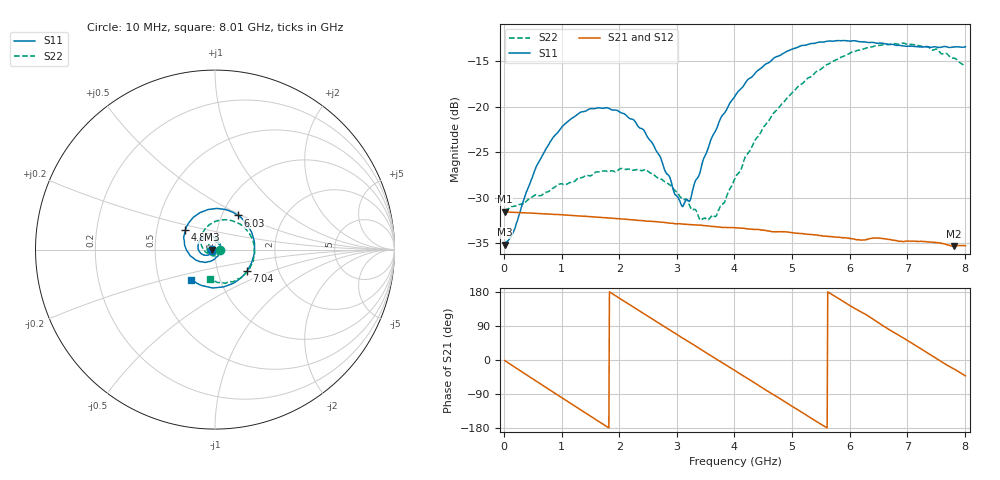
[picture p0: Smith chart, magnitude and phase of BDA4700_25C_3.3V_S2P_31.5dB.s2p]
!Agilent Technologies,E5071B,MY42404982,A.09.10
!Date: Mon Oct 20 18:16:19 2025
!Data & Calibration Information:
!Freq	S11:SOLT2(ON)	S21:SOLT2(ON)	S12:SOLT2(ON)	S22:SOLT2(ON)
# Hz S RI R 50
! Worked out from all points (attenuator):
!   801 points, 10 MHz to 8.01 GHz, reference 50 ohm
!   highest |S21| = -31.55 dB at 10 MHz (marker M1); lowest = -35.3 dB at 7.81 GHz (marker M2)
!   lowest |S11| = -35.1 dB at 10 MHz (marker M3), VSWR 1.04, Z = 48.3 - j0.0939 ohm
!   |S11| at or under -10 dB: start of sweep to end of sweep
!   |S22| runs from -32.5 to -13.0 dB; largest |S21 - S12| = 0.00037
!   S11 on the Smith chart (normalised r, x): 10 MHz: 0.97, -0.00; 4.87 GHz: 0.70, +0.16; 6.03 GHz: 1.19, +0.48; 7.04 GHz: 1.39, -0.35; 8.01 GHz: 0.73, -0.26
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1e7  -0.0175 -0.000972  0.0265 -0.00056  0.0264 -0.000587  0.0272 -0.000841
1.6e8  -0.0181 -0.00943  0.0252 -0.00737  0.0252 -0.00733  0.0273 -0.00771
5.4e8  -0.035 -0.0288  0.0153 -0.021  0.0153 -0.021  0.0163 -0.0283
7.6e8  -0.0517 -0.032  0.00641 -0.0249  0.00639 -0.0249  0.00204 -0.0339
1.35e9  -0.0937 0.00276  -0.0172 -0.0182  -0.0172 -0.0182  -0.0364 -0.0183
2.08e9  -0.0557 0.0727  -0.022 0.00995  -0.022 0.00995  -0.0303 0.0336
2.42e9  -0.0127 0.0736  -0.0128 0.0198  -0.0128 0.0198  -0.00543 0.0444
2.68e9  0.0156 0.0528  -0.0032 0.023  -0.00322 0.023  0.0126 0.0384
3.11e9  0.0279 -0.00569  0.0124 0.019  0.0122 0.019  0.0288 0.0111
3.24e9  0.021 -0.023  0.0159 0.0159  0.0159 0.0158  0.0276 0.00213
3.55e9  -0.0127 -0.0585  0.0213 0.00584  0.0213 0.00581  0.0132 -0.02
3.69e9  -0.0355 -0.0668  0.0219 0.000835  0.0219 0.00077  0.00167 -0.0252
4.01e9  -0.0957 -0.0623  0.0191 -0.0102  0.0191 -0.0101  -0.0308 -0.0259
4.37e9  -0.1537 -0.0113  0.00989 -0.0187  0.00987 -0.0187  -0.0663 0.00191
4.87e9  -0.1649 0.1099  -0.00688 -0.0194  -0.00674 -0.0193  -0.074 0.0774
5.35e9  -0.077 0.2086  -0.018 -0.0083  -0.0179 -0.00846  -0.0163 0.1464
6.03e9  0.1285 0.1901  -0.0147 0.0118  -0.0148 0.0117  0.1369 0.1443
6.68e9  0.2202 -0.000683  0.00301 0.0184  0.00303 0.0184  0.2193 0.000667
7.04e9  0.1789 -0.1194  0.0122 0.0136  0.0122 0.0135  0.1977 -0.0955
7.46e9  0.0571 -0.2053  0.0178 0.00268  0.0178 0.00261  0.1108 -0.1725
7.81e9  -0.0685 -0.2012  0.0157 -0.00685  0.0157 -0.00689  0.0182 -0.1838
8.01e9  -0.1311 -0.1683  0.0128 -0.0115  0.0129 -0.0114  -0.0294 -0.1637
